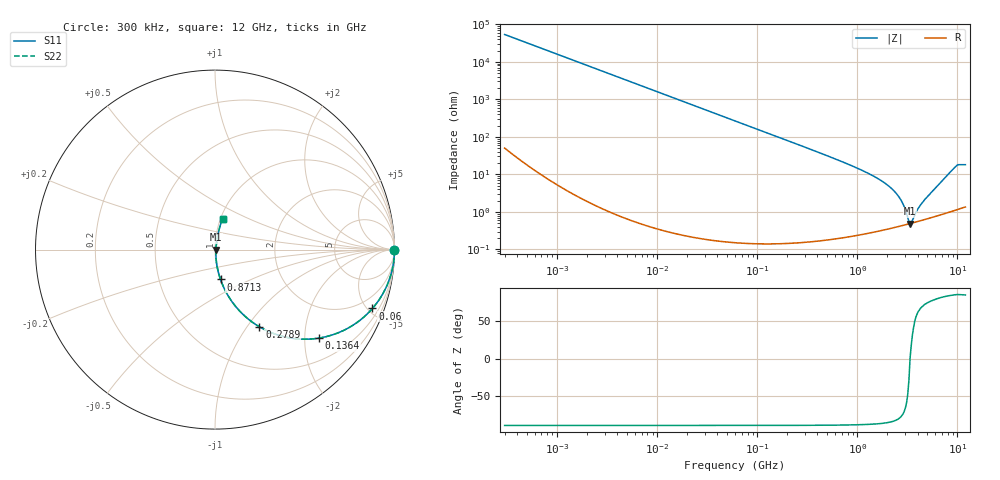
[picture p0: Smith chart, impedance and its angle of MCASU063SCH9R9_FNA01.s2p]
! MCASU063SCH9R9_FNA01  S-PARAMETER MODEL  ( General Type )
! Model Generated by TAIYO YUDEN Corporation (http://www.ty-top.com)
! Version 1.0
! TAIYO YUDEN Control No. 130801
! Copyright(c) 2013 TAIYO YUDEN CO.,LTD. All Rights Reserved.
! Product Description (link to TY-COMPAS)
! https://ds.yuden.co.jp/TYCOMPAS/or/detail?pn=MCASU063SCH9R9DFNA01&u=M
! Products Name : Multilayer Ceramic Capacitors
! Characteristics :
!  Capacitance : 9.9 pF , Rated Voltage : 50V , TCC : CH / C0H
!  Case Size : 0.6 x 0.3 / 0.024 x 0.012 [mm/inch] , Thickness : 0.3 / 0.012 [mm/inch]
!  (Conditions: Temperature = 25 degC , DC Bias Current/Voltage = 0A / 0V)
! External Node Assignments :
!  1  o---| |---o  2
! GND o---------o GND
! Frequency Range : 0.3MHz  -  12000MHz  [ 401 STEP ]
# MHz S RI R 50
! Freq[MHz].  S11 Real  S11 Imag  S21 Real  S21 Imag  S12 Real  S12 Imag  S22 Real  S22 Imag
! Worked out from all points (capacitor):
!   401 points, 300 kHz to 12 GHz, reference 50 ohm
!   read as one part in series: C = 9.91 pF near 316.3 kHz
!   lowest |Z| = 490 mohm at 3.365 GHz (marker M1)
!   series resonance near 3.362 GHz, so ESL is about 230 pH
!   S11 on the Smith chart (normalised r, x): 300 kHz: open; 60 MHz: 1.00, -5.35; 136.4 MHz: 1.00, -2.35; 278.9 MHz: 1.00, -1.14; 871.3 MHz: 1.00, -0.34; 12 GHz: 1.03, +0.36
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0.3  1 -0.00187  5.24e-06 0.00187  5.24e-06 0.00187  1 -0.00187
1.769972  0.9999 -0.011  0.000124 0.011  0.000124 0.011  0.9999 -0.011
10.44266  0.9958 -0.0647  0.00422 0.0647  0.00422 0.0647  0.9958 -0.0647
26.39317  0.9737 -0.16  0.0263 0.16  0.0263 0.16  0.9737 -0.16
60  0.8773 -0.3278  0.1227 0.3278  0.1227 0.3278  0.8773 -0.3278
136.3989  0.5801 -0.493  0.4199 0.493  0.4199 0.493  0.5801 -0.493
278.9009  0.247 -0.43  0.753 0.43  0.753 0.43  0.247 -0.43
353.9943  0.1685 -0.3725  0.8315 0.3725  0.8315 0.3725  0.1685 -0.3725
871.3074  0.0308 -0.1663  0.9692 0.1663  0.9692 0.1663  0.0308 -0.1663
1480.043  0.0104 -0.0864  0.9896 0.0864  0.9896 0.0864  0.0104 -0.0864
2088.533  0.00576 -0.0469  0.9942 0.0469  0.9942 0.0469  0.00576 -0.0469
2448.343  0.00487 -0.0306  0.9951 0.0306  0.9951 0.0306  0.00487 -0.0306
2722.03  0.00463 -0.0203  0.9954 0.0203  0.9954 0.0203  0.00463 -0.0203
2947.191  0.00461 -0.0126  0.9954 0.0126  0.9954 0.0126  0.00461 -0.0126
3190.978  0.00472 -0.00508  0.9953 0.00508  0.9953 0.00508  0.00472 -0.00508
3364.605  0.00487 8.51e-05  0.9951 -8.51e-05  0.9951 -8.51e-05  0.00487 8.51e-05
3547.679  0.00507 0.00312  0.9949 -0.00312  0.9949 -0.00312  0.00507 0.00312
4050.141  0.00569 0.011  0.9943 -0.011  0.9943 -0.011  0.00569 0.011
4502.883  0.00631 0.017  0.9937 -0.017  0.9937 -0.017  0.00631 0.017
8732.115  0.0252 0.1208  0.9748 -0.1208  0.9748 -0.1208  0.0252 0.1208
9968.853  0.0409 0.1682  0.9591 -0.1682  0.9591 -0.1682  0.0409 0.1682
12000  0.0439 0.1708  0.9561 -0.1708  0.9561 -0.1708  0.0439 0.1708
